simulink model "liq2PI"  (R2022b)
settings: Solver=ode45  StartTime=0.0  StopTime=500  FixedStep=1  RelTol=1e-6  EnableMultiTasking=on
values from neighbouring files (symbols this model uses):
  Ar = 6*25.4    (= 152.4)    [para2Kp.m]
  k1 = 0    [para2Kp.m]
  k12 = 38    [para2Kp.m]
  k2 = 11.5    [para2Kp.m]
  Kp = 10    [para2Kp.m]
  qmax = 90    [para2Kp.m]
  qmin = -85    [para2Kp.m]
undefined symbols (not defined in the file or in its folder): Ki
libraries: simulink x1

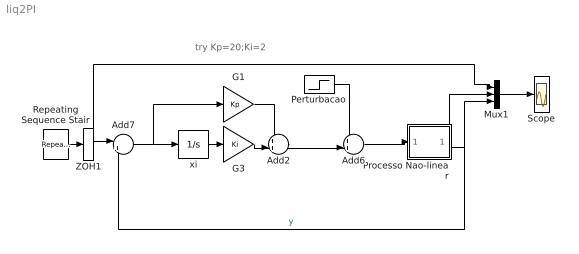
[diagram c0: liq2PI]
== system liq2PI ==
  note: try Kp=20;Ki=2
  Add2 : Sum  Inputs=++|
  Add6 : Sum  Inputs=++|
  Add7 : Sum  Inputs=|+-
  G1 : Gain  Gain=Kp
  G3 : Gain  Gain=Ki
  Mux1 : Mux  Inputs=3
  Perturbacao : Step  Time=350  After=200  SampleTime=0
  Processo Nao-linear : Subsystem
  Repeating Sequence Stair : simulink/Sources/Repeating Sequence Stair  OutValues=[2 5 12 5 2].'  tsamp=100  OutMin=[]  OutMax=[]  OutDataTypeStr=double  OutputDataTypeScalingMode=double  OutDataType=fixdt(0,8)  ConRadixGroup=Best Precision: Vector-wise  OutScaling=2^-12
  Scope : Scope
  ZOH1 : ZeroOrderHold
  xi : Integrator
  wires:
  Mux1/1 -> Scope/1
  Add2/1 -> Add6/2
  Processo Nao-linear/2(H2) -> Mux1/3, Add7/2  "y"
  Processo Nao-linear/1(H1) -> Mux1/2
  Perturbacao/1 -> Add6/1
  xi/1 -> G3/1
  G3/1 -> Add2/2
  G1/1 -> Add2/1
  Repeating Sequence Stair/1 -> ZOH1/1
  ZOH1/1 -> Add7/1, Mux1/1
  Add6/1 -> Processo Nao-linear/1(u)
  Add7/1 -> G1/1, xi/1

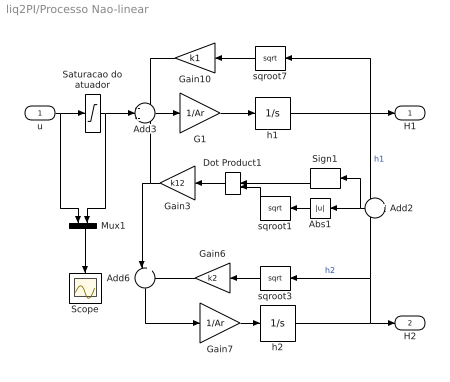
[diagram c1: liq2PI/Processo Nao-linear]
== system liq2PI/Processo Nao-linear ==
  u : Inport
  Abs1 : Abs
  Add2 : Sum  Inputs=+-
  Add3 : Sum  Inputs=-+-
  Add6 : Sum  Inputs=|+-
  Dot Product1 : DotProduct
  G1 : Gain  Gain=1/Ar
  Gain10 : Gain  Gain=k1
  Gain3 : Gain  Gain=k12
  Gain6 : Gain  Gain=k2
  Gain7 : Gain  Gain=1/Ar
  Mux1 : Mux  Inputs=2
  Saturacao do atuador : Saturate  UpperLimit=qmax  LowerLimit=qmin
  Scope : Scope
  Sign1 : Signum
  h1 : Integrator  LimitOutput=on  UpperSaturationLimit=16.5  LowerSaturationLimit=0
  h2 : Integrator  LimitOutput=on  UpperSaturationLimit=16.5  LowerSaturationLimit=0
  sqroot1 : Math  Operator=sqrt  SignedPower=on
  sqroot3 : Math  Operator=sqrt  SignedPower=on
  sqroot7 : Math  Operator=sqrt  SignedPower=on
  H1 : Outport
  H2 : Outport  Port=2
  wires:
  h1/1 -> Add2/1, H1/1, sqroot7/1  "h1"
  h2/1 -> Add2/2, sqroot3/1, H2/1  "h2"
  Saturacao do atuador/1 -> Add3/2, Mux1/2
  Add6/1 -> Gain7/1
  Gain10/1 -> Add3/1
  sqroot7/1 -> Gain10/1
  Gain6/1 -> Add6/2
  Gain7/1 -> h2/1
  sqroot3/1 -> Gain6/1
  G1/1 -> h1/1
  Gain3/1 -> Add6/1, Add3/3
  Add3/1 -> G1/1
  Dot Product1/1 -> Gain3/1
  sqroot1/1 -> Dot Product1/2
  Sign1/1 -> Dot Product1/1
  Abs1/1 -> sqroot1/1
  Add2/1 -> Abs1/1, Sign1/1
  u/1 -> Saturacao do atuador/1, Mux1/1
  Mux1/1 -> Scope/1
